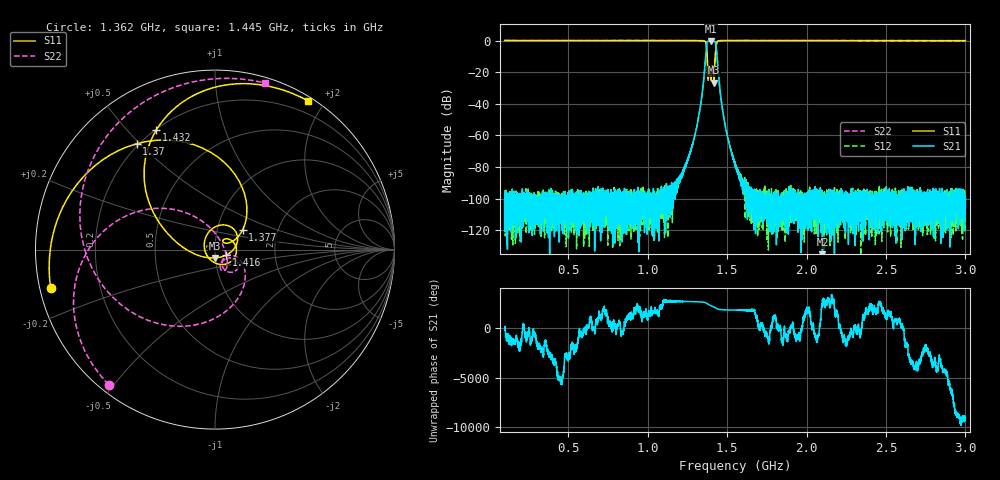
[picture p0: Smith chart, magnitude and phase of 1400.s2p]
# Hz S DB R 50
! Planar, S50180, 20087770, 20.1.2/1
! Date: 23.06.2021 14:43:00
! Data: Format (Calibration Info)
! Freq	S11:dB/Ang(F2)	S21:dB/Ang(F2)	S12:dB/Ang(F2)	S22:dB/Ang(F2)
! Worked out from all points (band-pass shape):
!   8991 points, 100 MHz to 3 GHz, reference 50 ohm
!   highest |S21| = -0.38 dB at 1.399 GHz (marker M1); lowest = -136.9 dB at 2.1 GHz (marker M2)
!   |S21| within 3 dB of the highest: 1.371 GHz to 1.431 GHz (59.71 MHz wide, 4.26 % of centre)
!   lowest |S11| = -26.7 dB at 1.418 GHz (marker M3), VSWR 1.10, Z = 49.6 - j4.6 ohm
!   |S11| at or under -10 dB: 1.375 GHz to 1.426 GHz (50.76 MHz wide, 3.62 % of centre)
!   |S22| runs from -26.1 to 0.0 dB; largest |S21 - S12| = 0.0024
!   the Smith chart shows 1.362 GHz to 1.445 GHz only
!   S11 on the Smith chart (normalised r, x): 1.362 GHz: 0.03, -0.11; 1.37 GHz: 0.19, +0.49; 1.377 GHz: 1.33, +0.31; 1.416 GHz: 1.13, -0.07; 1.432 GHz: 0.20, +0.60; 1.445 GHz: 0.05, +1.80
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1e8  0.02 154.0  -104.83 -167.4  -103.29 4.3  0.01 150.2
3.125806e8  -0.03 104.1  -109.84 -56.8  -105.63 -81.3  0.00 95.3
5.835484e8  -0.01 54.8  -103.07 157.8  -96.26 -99.9  0.01 45.6
1.066774e9  -0.00 -9.9  -102.76 17.8  -93.82 -62.1  0.04 -15.0
1.244194e9  -0.01 -40.4  -77.03 -131.6  -77.40 -126.2  0.04 -41.2
1.336452e9  -0.10 -92.1  -38.77 -177.7  -38.77 -177.7  -0.03 -79.6
1.362258e9  -0.53 -166.9  -14.33 119.3  -14.33 119.2  -0.38 -128.2
1.369677e9  -2.69 126.5  -4.88 62.1  -4.89 62.1  -2.51 -174.0
1.376774e9  -14.38 35.8  -0.73 -19.5  -0.74 -19.6  -14.71 116.2
1.388387e9  -18.54 4.7  -0.45 -118.9  -0.46 -119.0  -17.97 -62.5
1.39871e9  -25.20 -150.7  -0.38 167.8  -0.39 167.7  -22.41 -49.1
1.407742e9  -16.50 65.2  -0.47 105.0  -0.48 104.9  -15.81 -37.5
1.416452e9  -23.07 -25.0  -0.43 41.2  -0.43 41.1  -21.56 -62.6
1.418387e9  -26.70 -91.8  -0.44 25.6  -0.44 25.5  -23.26 -37.0
1.432258e9  -2.58 116.1  -4.62 -116.3  -4.62 -116.4  -2.96 -176.0
1.444839e9  -0.20 58.1  -20.37 158.5  -20.38 158.4  -0.28 73.3
1.470968e9  -0.04 19.3  -43.27 110.0  -43.29 109.7  -0.05 17.3
1.55e9  -0.02 -15.0  -78.09 70.3  -78.21 75.0  0.03 -20.7
2.033548e9  -0.04 -70.1  -99.21 -139.7  -102.30 -147.8  -0.01 -72.0
2.100323e9  -0.02 -75.3  -136.94 -5.8  -120.58 19.8  0.02 -77.0
2.516774e9  -0.07 -106.8  -97.46 172.6  -100.75 173.1  -0.05 -105.6
3e9  -0.10 -142.4  -99.24 -162.6  -97.13 -19.4  -0.09 -138.7
